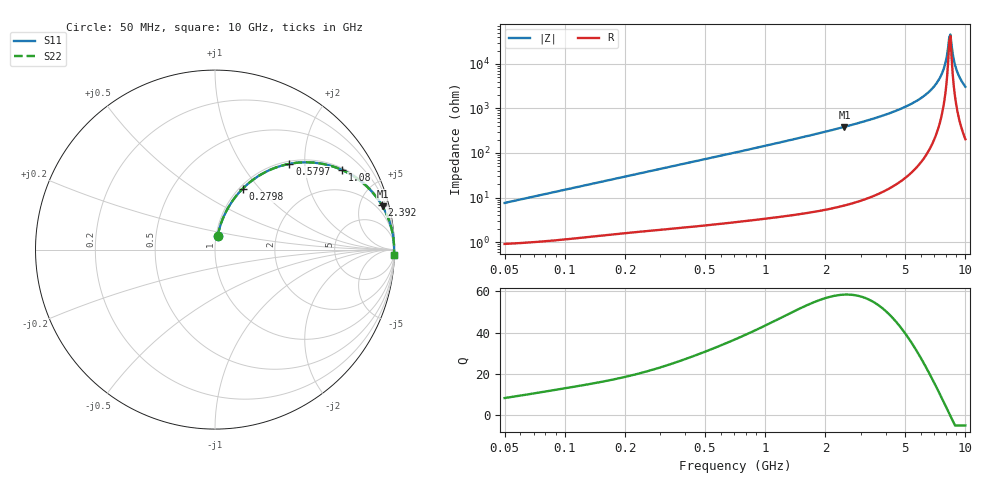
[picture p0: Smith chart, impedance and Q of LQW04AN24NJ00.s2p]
!Murata Part Number: LQW04AN24NJ00
!These Parameters are Measured in Series Mode Connection
!  o--[Z]--o
!Port1  Port2
!  o-------o
!Freq. Start=50[MHz] Stop=10[GHz], 401[Steps]
# Hz S RI R 50
!Freq.(Hz)	S 11(Real)	S 11(Imag)	S 21(Real)	S 21(Imag)	S 12(Real)	S 12(Imag)	S 22(Real)	S 22(Imag)
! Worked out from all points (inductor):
!   401 points, 50 MHz to 10 GHz, reference 50 ohm
!   read as one part in series: L = 23.8 nH near 51.34 MHz
!   highest Q = 58.4 at 2.489 GHz (marker M1), where L = 24.7 nH
!   self-resonance near 8.307 GHz
!   S11 on the Smith chart (normalised r, x): 50 MHz: 1.02, +0.15; 279.8 MHz: 1.04, +0.81; 579.7 MHz: 1.05, +1.67; 1.08 GHz: 1.07, +3.13; 2.392 GHz: 1.13, +7.37; 10 GHz: 5, -61
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5e7  0.0145 0.0734  0.9855 -0.0734  0.9855 -0.0734  0.0145 0.0734
1.214486e8  0.0426 0.1702  0.9574 -0.1702  0.9574 -0.1702  0.0426 0.1702
2.797723e8  0.1533 0.3385  0.8467 -0.3385  0.8467 -0.3385  0.1533 0.3385
2.949953e8  0.1661 0.351  0.8339 -0.351  0.8339 -0.351  0.1661 0.351
5.796908e8  0.4146 0.4778  0.5854 -0.4778  0.5854 -0.4778  0.4146 0.4778
7.071068e8  0.5101 0.4864  0.4899 -0.4864  0.4899 -0.4864  0.5101 0.4864
1.080357e9  0.7065 0.4444  0.2935 -0.4444  0.2935 -0.4444  0.7065 0.4444
1.717543e9  0.8618 0.336  0.1382 -0.336  0.1382 -0.336  0.8618 0.336
2.391784e9  0.9277 0.2505  0.0723 -0.2505  0.0723 -0.2505  0.9277 0.2505
2.488741e9  0.9336 0.2406  0.0664 -0.2406  0.0664 -0.2406  0.9336 0.2406
4.171863e9  0.9813 0.1257  0.0187 -0.1257  0.0187 -0.1257  0.9813 0.1257
5.657692e9  0.9931 0.0686  0.00691 -0.0686  0.00691 -0.0686  0.9931 0.0686
6.901252e9  0.9968 0.0337  0.00318 -0.0337  0.00318 -0.0337  0.9968 0.0337
7.672705e9  0.9978 0.0154  0.00224 -0.0154  0.00224 -0.0154  0.9978 0.0154
7.878683e9  0.9979 0.0108  0.00212 -0.0108  0.00212 -0.0108  0.9979 0.0108
8.198065e9  0.998 0.00383  0.00202 -0.00383  0.00202 -0.00383  0.998 0.00383
8.307378e9  0.998 0.0015  0.00201 -0.0015  0.00201 -0.0015  0.998 0.0015
8.530394e9  0.998 -0.00318  0.00203 0.00318  0.00203 0.00318  0.998 -0.00318
8.876195e9  0.9979 -0.0103  0.00214 0.0103  0.00214 0.0103  0.9979 -0.0103
9.114482e9  0.9977 -0.0151  0.00228 0.0151  0.00228 0.0151  0.9977 -0.0151
9.610418e9  0.9973 -0.0248  0.00272 0.0248  0.00272 0.0248  0.9973 -0.0248
1e10  0.9968 -0.0323  0.0032 0.0323  0.0032 0.0323  0.9968 -0.0323
